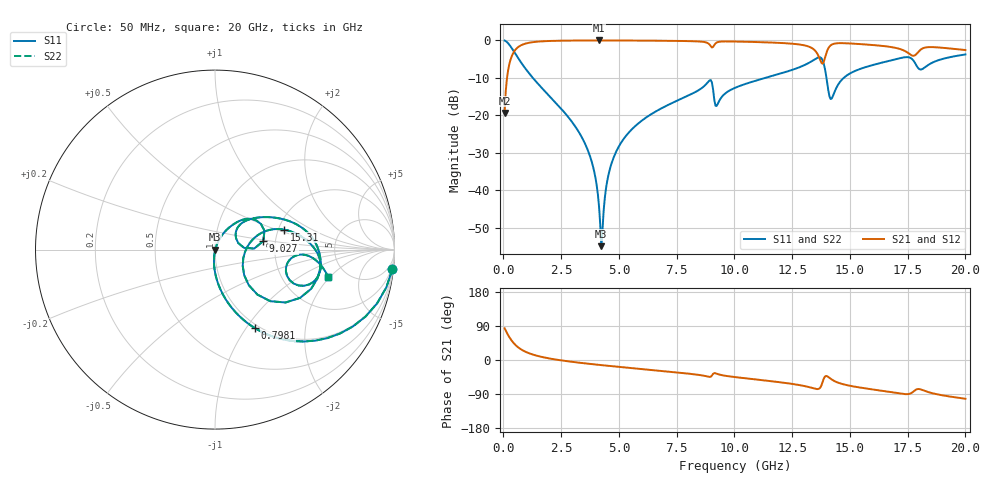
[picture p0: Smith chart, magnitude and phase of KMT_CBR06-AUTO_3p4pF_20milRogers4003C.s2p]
! Data measured by Modelithics Inc. support@modelithics.com 813-866-6335
! KEMET CBR06-AUTO 3.4pF, Pad Width= 0.851mm, Pad Length= 0.64mm, Pad Gap= 0.62mm, 20mil Rogers 4003C substrate Data, January 2022
# hz S ma R 50
! 2 Port Network Data from SP1.SP block
! freq  magS11  angS11  magS21  angS21  magS12  angS12  magS22  angS22
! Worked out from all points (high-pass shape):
!   401 points, 50 MHz to 20 GHz, reference 50 ohm
!   highest |S21| = -0.02 dB at 4.14 GHz (marker M1); lowest = -19.4 dB at 50 MHz (marker M2)
!   |S21| within 3 dB of the highest: 459.4 MHz to 13.53 GHz (13.07 GHz wide, 187 % of centre); 14 GHz to 17.43 GHz (3.434 GHz wide, 21.8 % of centre)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
!   lowest |S11| = -55.0 dB at 4.239 GHz (marker M3), VSWR 1.00, Z = 50.2 - j0.0696 ohm
!   |S11| at or under -10 dB: 1.271 GHz to 11.35 GHz (10.08 GHz wide, 160 % of centre); 13.98 GHz to 14.73 GHz (751.5 MHz wide, 5.23 % of centre)
!   |S22| runs from -55.0 to -0.1 dB; largest |S21 - S12| = 0
!   S11 on the Smith chart (normalised r, x): 50 MHz: 1, -18; 798.1 MHz: 0.95, -1.09; 9.027 GHz: 1.72, +0.18; 15.31 GHz: 2.15, +0.57; 20 GHz: 3.62, -1.92
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5e7  0.9942 -6.3  0.1072 83.7  0.1072 83.7  0.9942 -6.3
2.99375e8  0.8386 -33.9  0.5439 56.0  0.5439 56.0  0.8386 -33.9
7.98125e8  0.4892 -63.2  0.8712 26.7  0.8712 26.7  0.4892 -63.2
3.391625e9  0.05093 -96.1  0.997 -7.9  0.997 -7.9  0.05093 -96.1
3.890375e9  0.01993 -96.4  0.998 -11.3  0.998 -11.3  0.01993 -96.4
4.13975e9  0.005997 -86.0  0.9981 -12.9  0.9981 -12.9  0.005997 -86.0
4.2395e9  0.001784 -22.9  0.9981 -13.5  0.9981 -13.5  0.001784 -22.9
4.53875e9  0.01559 67.9  0.9979 -15.4  0.9979 -15.4  0.01559 67.9
4.93775e9  0.03549 69.1  0.9973 -17.8  0.9973 -17.8  0.03549 69.1
6.73325e9  0.1188 60.6  0.9902 -28.2  0.9902 -28.2  0.1188 60.6
9.0275e9  0.2731 10.0  0.8045 -40.8  0.8045 -40.8  0.2731 10.0
9.227e9  0.133 28.0  0.9344 -36.1  0.9344 -36.1  0.133 28.0
1.0025e10  0.2325 43.3  0.9657 -45.1  0.9657 -45.1  0.2325 43.3
1.336662e10  0.5316 9.4  0.7856 -73.8  0.7856 -73.8  0.5316 9.4
1.366588e10  0.5956 -10.0  0.5946 -75.7  0.5946 -75.7  0.5956 -10.0
1.386538e10  0.4915 -36.8  0.5143 -49.7  0.5143 -49.7  0.4915 -36.8
1.42145e10  0.1677 -4.3  0.8782 -51.5  0.8782 -51.5  0.1677 -4.3
1.531175e10  0.4013 16.1  0.8981 -71.4  0.8981 -71.4  0.4013 16.1
1.670825e10  0.5341 3.3  0.8218 -84.2  0.8218 -84.2  0.5341 3.3
1.745638e10  0.5977 -10.6  0.7003 -90.2  0.7003 -90.2  0.5977 -10.6
1.805488e10  0.4079 -13.8  0.7492 -77.4  0.7492 -77.4  0.4079 -13.8
2e10  0.6496 -13.7  0.7436 -102.2  0.7436 -102.2  0.6496 -13.7
